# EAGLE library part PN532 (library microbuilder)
PN532 - Near Field Communication (NFC) controller Highly integrated transceiver module for contactless communication at 13.56 MHz (14443A/MIFARE, FeliCa, I4443B)
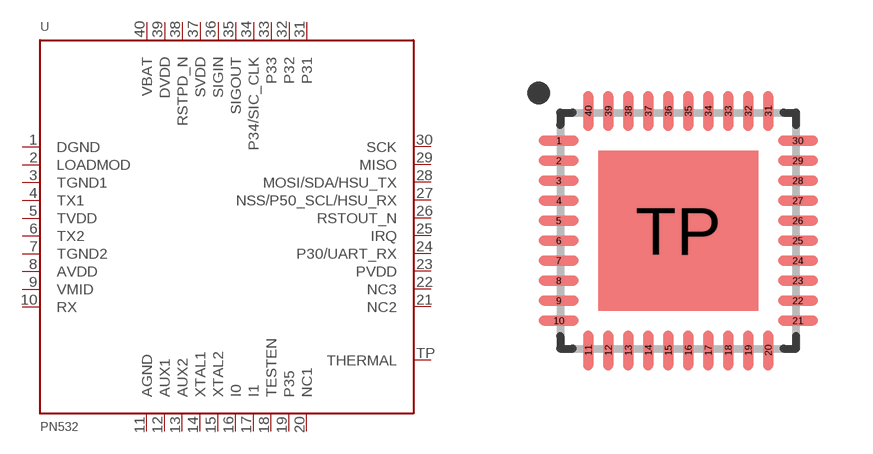
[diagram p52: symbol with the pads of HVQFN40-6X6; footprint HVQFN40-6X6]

Designator prefix U

## PN532  [HVQFN40-6X6]
1  DGND
2  LOADMOD
3  TGND1
4  TX1
5  TVDD
6  TX2
7  TGND2
8  AVDD
9  VMID
10  RX
11  AGND
12  AUX1
13  AUX2
14  XTAL1
15  XTAL2
16  I0
17  I1
18  TESTEN
19  P35
20  NC1
21  NC2
22  NC3
23  PVDD
24  P30/UART_RX
25  IRQ
26  RSTOUT_N
27  NSS/P50_SCL/HSU_RX
28  MOSI/SDA/HSU_TX
29  MISO
30  SCK
31  P31
32  P32
33  P33
34  P34/SIC_CLK
35  SIGOUT
36  SIGIN
37  SVDD
38  RSTPD_N
39  DVDD
40  VBAT
TP  THERMAL

## Footprint HVQFN40-6X6 (pad centres in mm)
HVQFN40 Plastic thermal enhanced very thin quad flat package; 40 terminals; body 6x6x0.85 mm;
smd 1 x 0.25: 1 -2.99,2.25; 2 -2.99,1.75; 3 -2.99,1.25; 4 -2.99,0.75; 5 -2.99,0.25; 6 -2.99,-0.25; 7 -2.99,-0.75; 8 -2.99,-1.25; 9 -2.99,-1.75; 10 -2.99,-2.25; 21 2.99,-2.25; 22 2.99,-1.75; 23 2.99,-1.25; 24 2.99,-0.75; 25 2.99,-0.25; 26 2.99,0.25; 27 2.99,0.75; 28 2.99,1.25; 29 2.99,1.75; 30 2.99,2.25
smd 0.25 x 1: 11 -2.25,-2.99; 12 -1.75,-2.99; 13 -1.25,-2.99; 14 -0.75,-2.99; 15 -0.25,-2.99; 16 0.25,-2.99; 17 0.75,-2.99; 18 1.25,-2.99; 19 1.75,-2.99; 20 2.25,-2.99; 31 2.25,2.99; 32 1.75,2.99; 33 1.25,2.99; 34 0.75,2.99; 35 0.25,2.99; 36 -0.25,2.99; 37 -0.75,2.99; 38 -1.25,2.99; 39 -1.75,2.99; 40 -2.25,2.99
smd 4 x 4: TP 0,0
